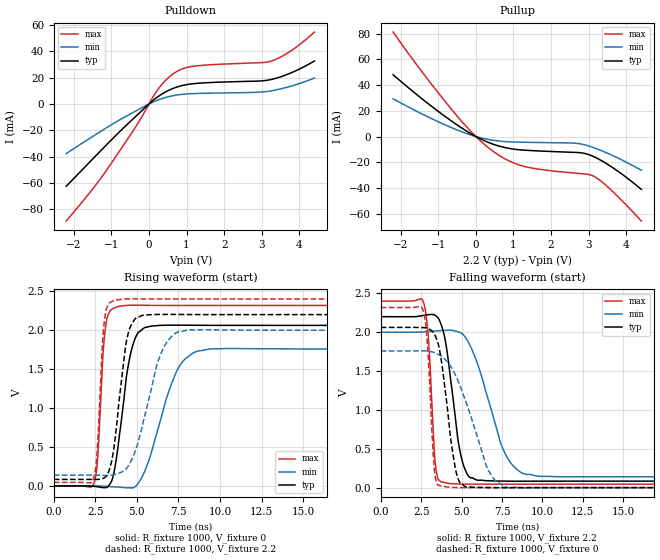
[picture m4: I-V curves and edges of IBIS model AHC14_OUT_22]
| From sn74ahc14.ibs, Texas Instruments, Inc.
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[Model]   AHC14_OUT_22
Model_type  Output
Vref =   0
Rref =   1000
Cref =   50p
Vmeas =   1.1
| variable   typ   min   max
C_comp   2.98pF   1.56pF   4.52pF
| C_pullup   2.80pF   1.56pF   3.52pF
| C_pulldown   3.16pF   1.77pF   4.52pF
[Temperature Range]   40   100   -40
| Ambient temperature   25   85   -40
[Voltage range]   2.2   2   2.4
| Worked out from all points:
|   slope of the pulldown table from 0 to 0.33 V, typ, clamps not added: 45.1 ohm
|   slope of the pullup table from 0 to 0.33 V, typ, clamps not added: 72.7 ohm
|   rising waveform, R_fixture 1000, V_fixture 0: 20-80 % time 767ps typ, 1.5ns min, 349ps max; typ from 0 V to 2.06 V
|   falling waveform, R_fixture 1000, V_fixture 2.2: 20-80 % time 783ps typ, 1.61ns min, 351ps max; typ from 2.2 V to 0.083 V
|   rising waveform, R_fixture 1000, V_fixture 2.2: 20-80 % time 677ps typ, 1.32ns min, 330ps max; typ from 0.083 V to 2.2 V
|   falling waveform, R_fixture 1000, V_fixture 0: 20-80 % time 742ps typ, 1.71ns min, 353ps max; typ from 2.06 V to 0 V
[Pulldown]
| AHC14_OUT_22
|   Voltage   I(typ)   I(min)   I(max)
-2.2V     -62.5mA    -37.71mA   -88.97mA
-1.57V    -43.98mA   -26.01mA   -67.23mA
-1.155V   -31.79mA   -18.52mA   -51.42mA
-380mV    -10.19mA   -5.783mA   -18.54mA
10mV      264.1uA    144.1uA    536.1uA
295mV     6.674mA    3.624mA    13.19mA
610mV     11.5mA     6.157mA    22.25mA
875mV     13.99mA    7.339mA    26.61mA
1.185V    15.46mA    7.929mA    28.73mA
3.235V    18.57mA    9.958mA    32.54mA
3.76V     23.49mA    13.45mA    40.15mA
4.4V      32.72mA    19.75mA    54.74mA
[Pullup]
| AHC14_OUT_22
|   Voltage   I(typ)   I(min)   I(max)
-2.2V     48mA       29.29mA    81.17mA
-1.415V   28.89mA    17.28mA    49.61mA
-575mV    10.55mA    6.012mA    18.55mA
-50mV     801.5uA    426.7uA    1.459mA
395mV     -5.276mA   -2.621mA   -10.1mA
835mV     -8.961mA   -4.058mA   -18.26mA
1.28V     -10.57mA   -4.458mA   -23.18mA
2.635V    -12.33mA   -5.195mA   -28.44mA
2.885V    -13.1mA    -6.389mA   -29.05mA
3.12V     -15.48mA   -8.519mA   -30.68mA
3.585V    -23.12mA   -14.08mA   -41.24mA
4.4V      -41.05mA   -26.22mA   -65.64mA
[Ramp]
| AHC14_OUT_22
| variable   typ   min   max
dV/dt_r   1.25/8.57E-10   1.07/1.59E-09   1.40/3.77E-10
dV/dt_f   1.29/8.58E-10   1.13/1.71E-09   1.43/3.60E-10
R_load = 1000
[Rising Waveform]
| AHC14_OUT_22
R_fixture =   1000
C_fixture =   0
L_fixture =   0
V_fixture =   0
V_fixture_min = 0
V_fixture_max = 0
|   Time   V(typ)   V(min)   V(max)
0s        865.9pV    1.52nV     445.3pV
2.405ns   -5.276mV   603.8uV    32.87mV
2.63ns    -11.19mV   660.7uV    339.7mV
3.14ns    -21.41mV   -5.193mV   2.079V
3.975ns   694.6mV    -17.24mV   2.308V
4.49ns    1.56V      -24.55mV   2.319V
5.06ns    1.964V     28.62mV    2.32V
7.395ns   2.064V     1.475V     2.318V
8.75ns    2.063V     1.736V     2.318V
50ns      2.062V     1.758V     2.318V
[Falling Waveform]
| AHC14_OUT_22
R_fixture =   1000
C_fixture =   0
L_fixture =   0
V_fixture =   2.2
V_fixture_min = 2
V_fixture_max = 2.4
|   Time   V(typ)   V(min)   V(max)
0s        2.2V       2V         2.4V
2.645ns   2.216V     2.004V     2.387V
2.94ns    2.226V     2.01V      1.953V
3.375ns   2.216V     2.016V     316.8mV
3.76ns    2.084V     2.021V     70.36mV
4.98ns    394.2mV    1.989V     45.04mV
5.975ns   95.93mV    1.6V       44.34mV
7.565ns   83.51mV    495.6mV    44.73mV
8.985ns   82.37mV    170.9mV    44.9mV
50ns      83.34mV    138.6mV    44.92mV
[Rising Waveform]
| AHC14_OUT_22
R_fixture =   1000
C_fixture =   0
L_fixture =   0
V_fixture =   2.2
V_fixture_min = 2
V_fixture_max = 2.4
|   Time   V(typ)   V(min)   V(max)
0s        83.34mV    138.6mV    44.92mV
2.365ns   83.59mV    138.2mV    81.74mV
2.595ns   83.25mV    137.8mV    404.6mV
3.045ns   105.2mV    134.9mV    2.121V
3.785ns   788.3mV    153mV      2.387V
4.31ns    1.785V     209.2mV    2.4V
4.82ns    2.125V     401.1mV    2.402V
6.46ns    2.203V     1.707V     2.4V
7.975ns   2.201V     2V         2.4V
50ns      2.2V       2V         2.4V
[Falling Waveform]
| AHC14_OUT_22
R_fixture =   1000
C_fixture =   0
L_fixture =   0
V_fixture =   0
V_fixture_min = 0
V_fixture_max = 0
|   Time   V(typ)   V(min)   V(max)
0s        2.062V     1.758V     2.318V
2.625ns   2.059V     1.76V      2.28V
2.895ns   2.05V      1.758V     1.828V
3.315ns   1.978V     1.737V     233.8mV
3.685ns   1.717V     1.7V       20.48mV
4.65ns    214.2mV    1.435V     1.448mV
5.325ns   5.384mV    1.072V     -393.7uV
6.68ns    558.5uV    215.3mV    -279.7uV
7.955ns   -757.2uV   -2.436mV   -81.6uV
50ns      2.008nV    13.69nV    -15.58nV
